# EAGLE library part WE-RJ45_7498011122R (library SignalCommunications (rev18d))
Order Code 7498011122R Design SMD xBase-T 10/100 Base-T Ports 1x1 Application Standard Tab Position Up LED (Left-Right) YELLOW-GREEN EMI Fingers Yes Details see: http://katalog.we-online.de/en/pbs/WE-LAN_RJ45/7498011122R? Updated by Yingchun Shan 2016-08-23 2014 (C) Würth Elektronik
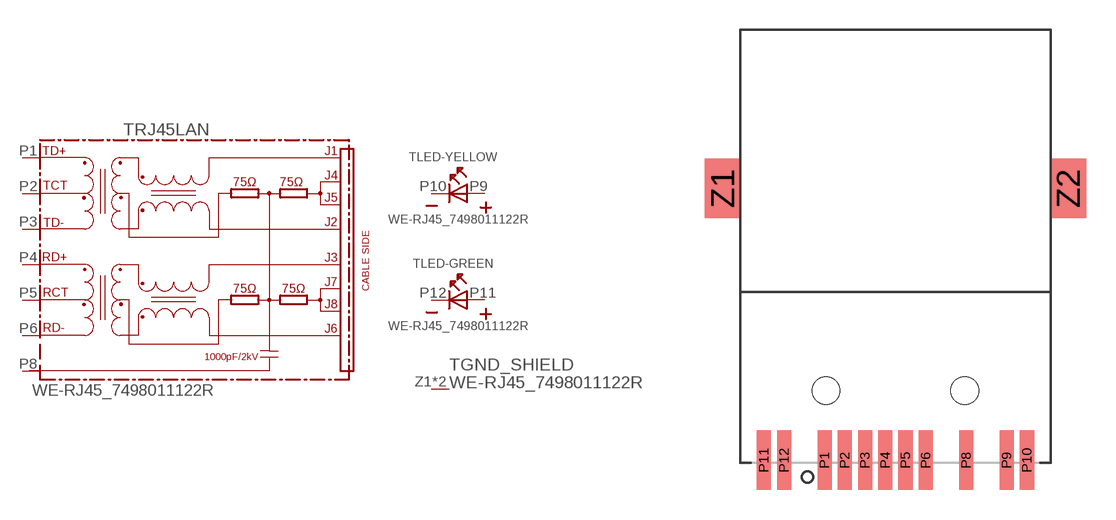
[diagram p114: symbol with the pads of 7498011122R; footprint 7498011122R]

Designator prefix T; gates RJ45LAN=74990X-THT-10/100-T LED-YELLOW=LED2PIN LED-GREEN=LED2PIN GND_SHIELD=GND_PIN

## WE-RJ45_7498011122R (COMPANY-URL: http://www.we-online.de; CREATED-BY: Christin Zierenner; CREATED-DATE: AUG 2012; DATASHEET-URL: http://katalog.we-online.de/kataloge/eisos/media/pdf/7498011122R.pdf; MANUFACTURER: Würth Elektronik eiSos GmbH)  [7498011122R]
P1  RJ45LAN:TD+
P2  RJ45LAN:TCT
P3  RJ45LAN:TD-
P4  RJ45LAN:RD+
P5  RJ45LAN:RCT
P6  RJ45LAN:RD-
P8  RJ45LAN:8
P9  LED-YELLOW:A  pas
P10  LED-YELLOW:K  pas
P11  LED-GREEN:A  pas
P12  LED-GREEN:K  pas
Z1  GND_SHIELD:1  pwr
Z2  GND_SHIELD:1  pwr

## Footprint 7498011122R (pad centres in mm)
MAX HEIGHT=11.30mm PORTS----1X1 LED --Yes
smd 0.71 x 3: P1 -3.57,-3.5; P2 -2.55,-3.5; P3 -1.53,-3.5; P4 -0.51,-3.5; P5 0.51,-3.5; P6 1.53,-3.5; P8 3.57,-3.5; P9 5.61,-3.5; P10 6.63,-3.5; P11 -6.63,-3.5; P12 -5.61,-3.5
smd 1.8 x 3: Z1 -8.71,10.2; Z2 8.71,10.2
hole 1.4 at -3.5,0
hole 1.4 at 3.5,0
